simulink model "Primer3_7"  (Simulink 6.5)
settings: Solver=ode23t  StartTime=0.0  StopTime=5  RelTol=1e-3
undefined symbols (not defined in the file or in its folder): blocks, Continuous, powergui, ZData
libraries: powerlib x3, powerlib_extras x2

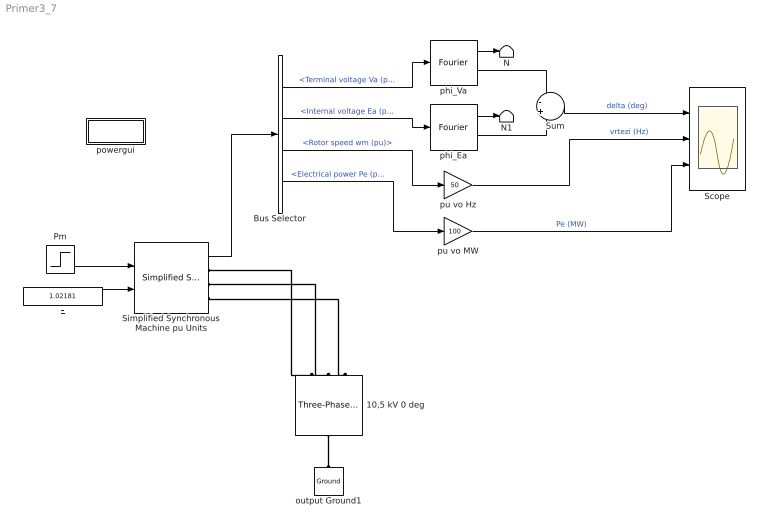
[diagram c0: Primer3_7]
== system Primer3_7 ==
  10,5 kV 0 deg : powerlib/Electrical Sources/Three-Phase Programmable Voltage Source  Orientation=up  DialogController=PMDialogs.PMDefaultMaskDlg  SystemSampleTime=-1  PositiveSequence="[10.5e3 0  50]"  VariationEntity=None  VariationType=Step  VariationStep=-0.5  VariationRate=10  VariationMagnitude=0.3  VariationFrequency=2  VariationTiming=[0.1 1.2]  VariationPhaseA=off  Amplitudes=[1 0.8 1.2 1.0]  TimeValues=[0 0.1 0.15 0.2]  HarmonicGeneration=off  HarmonicA=[3 0.2 -25 0]  HarmonicB="[2 0.15  35 2]"  Timing="[0.05  3]"
  Bus Selector : BusSelector  OutputSignals=Terminal voltage Va (pu),Internal voltage Ea (pu),Rotor speed wm (pu),Electrical power Pe (pu)
  E : Constant  Value=1.02181  OutDataType=sfix(16)  ConRadixGroup=Use specified scaling  OutScaling=2^0  SampleTime=inf  FramePeriod=inf
  N : Terminator
  N1 : Terminator
  Pm : Step  Time=0.5  Before=0.5  After=0.6  SampleTime=0
  Scope : Scope  NumInputPorts=3
  Simplified Synchronous Machine pu Units : powerlib/Machines/Simplified Synchronous Machine pu Units  DialogController=PMDialogs.PMDefaultMaskDlg  SystemSampleTime=-1  ConnectionType=3-wire Y  NominalParameters=[100e6 10.5e3 50]  Mechanical=[6 20 1]  InternalRL="[0  0.3+0.12]"  InitialConditions=[0 11.8598 0.5 0.5 0.5 0 -120 120]  Units=0  LoadFlowParameters=[1 50000000 0 0 0]
  Sum : Sum  Inputs=-+
  output Ground1 : powerlib/Elements/Ground  Orientation=down  DialogController=PMDialogs.PMDefaultMaskDlg  PhysicalDomain=powersysdomain  SubClassName=unknown  LeftPortType=p1  RightPortType=p1  LConnTagsString=a
  phi_Ea : powerlib_extras/Measurements/Fourier  DialogController=PMDialogs.PMDefaultMaskDlg  SystemSampleTime=-1  f1=50  n=1
  phi_Va : powerlib_extras/Measurements/Fourier  DialogController=PMDialogs.PMDefaultMaskDlg  SystemSampleTime=-1  f1=50  n=1
  powergui : Subsystem  AncestorBlock=powerlib/powergui  InitFcn=powergui( 'InitFcn_Callback' , gcb , 0 , [ ] );  mask(PSB option menu block){SimulationMode=Continuous, SampleTime=50e-6, echomessages=off, RestoreLinks=warning, x0status=blocks, Frange=[0:2:500], Ylog=off, Xlog=on, ShowGrid=off, save=off, variable=ZData, structure=, ZoomFFT=on, StartTime=0.0, cycles=1, DisplayStyle=1, fundamental=60, FreqAxis=off, MaxFrequency=1000, frequencyindice=50, frequencyindicesteady=1, RmsSteady=1, display=off, Ts=0, frequency=60, methode=off, HookPort=off, Interpol=off}
      mask prompts: SimulationMode "Simulation mode"; SampleTime "Sample time Ts (when simulation mode is Discrete) (s)"; echomessages "Echo  Messages"; RestoreLinks "Restore disabled links"; x0status "Initial electrical states status"; Frange "Impedance tool: Frequency Range"; Ylog "Impedance tool: Log impedance"; Xlog "Impedance tool: log Frequency"; ShowGrid "Impedance tool: grid"; save "Impedance tool: Save Data To Workspace"; variable "Impedance tool: Variable Name"; structure "Structure Name (PSBFFTSCOPE)"; ZoomFFT "ZoomFFT (PSBFFTSCOPE)"; StartTime "Start Time (PSBFFTSCOPE)"; cycles "Cycles (PSBFFTSCOPE)"; DisplayStyle "Display style (PSBFFTSCOPE)"; fundamental "Fundamental (PSBFFTSCOPE)"; FreqAxis "Frequency Axis (PSBFFTSCOPE)"; MaxFrequency "Max Frequency (PSBFFTSCOPE)"; frequencyindice "Load flow frequency (Hz)"; frequencyindicesteady "Frequency indice (STEADYSTATE)"; RmsSteady "RMS display (STEADYSTATE)"; display "Display Results"; Ts "OBSOLETE 1"; frequency "Phasor frequency (Hz)"; methode "Phasor simulation"; HookPort "Hook port"; Interpol "Interpolate"
      mask init:
      | powerlibroot = which('powersysdomain');
      | PSBroot = powerlibroot(1:end-16);
      | %
      | switch SimulationMode
      | 	case 1
      | 		message=sprintf('Continuous');
      | 	case 2
      |         SampleTimeeval=evalin('base',SampleTime,'NaN');
      |         if isnan(SampleTimeeval)
      |             message=sprintf('Warning !!,\nUndefined sample time');
      |         else
      |             message=sprintf('Discrete,\nTs = %.4g s.',SampleTimeeval);
      |         end
      | 	case 3
      | 		message=sprintf('Phasors');
      | end
      | if strcmp(bdroot,'powerlib')
      |   message='powergui';
      | end
      | power_initmask();
  pu vo Hz : Gain  Gain=50
  pu vo MW : Gain  Gain=100
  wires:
  E/1 -> Simplified Synchronous Machine pu Units/2
  Pm/1 -> Simplified Synchronous Machine pu Units/1
  phi_Va/2 -> Sum/1
  phi_Ea/2 -> Sum/2
  Sum/1 -> Scope/1  "delta (deg)"
  phi_Va/1 -> N/1
  phi_Ea/1 -> N1/1
  Bus Selector/1 -> phi_Va/1  "<Terminal voltage Va (pu)>"
  Bus Selector/2 -> phi_Ea/1  "<Internal voltage Ea (pu)>"
  Simplified Synchronous Machine pu Units/1 -> Bus Selector/1
  Bus Selector/3 -> pu vo Hz/1  "<Rotor speed wm (pu)>"
  pu vo Hz/1 -> Scope/2  "vrtezi (Hz)"
  Bus Selector/4 -> pu vo MW/1  "<Electrical power Pe (pu)>"
  pu vo MW/1 -> Scope/3  "Pe (MW)"
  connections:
  output Ground1/LConn1 -- 10,5 kV 0 deg/LConn1
  Simplified Synchronous Machine pu Units/RConn3 -- 10,5 kV 0 deg/RConn3
  Simplified Synchronous Machine pu Units/RConn2 -- 10,5 kV 0 deg/RConn2
  Simplified Synchronous Machine pu Units/RConn1 -- 10,5 kV 0 deg/RConn1

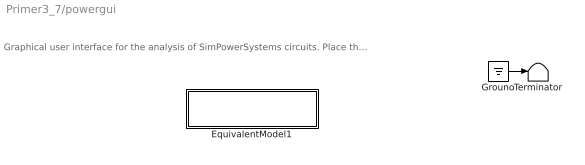
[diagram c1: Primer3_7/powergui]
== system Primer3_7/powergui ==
  note: Graphical user interface for the analysis of SimPowerSystems circuits. Place the Powergui block in the top-level of your model and double-click on it to open the GUI.
  EquivalentModel1 : Subsystem
  Ground : Ground
  Terminator : Terminator
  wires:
  Ground/1 -> Terminator/1

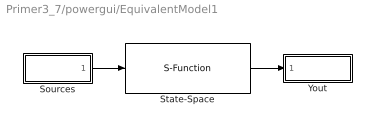
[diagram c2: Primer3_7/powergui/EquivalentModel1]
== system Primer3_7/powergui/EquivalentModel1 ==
  Sources : Subsystem
  State-Space : S-Function  FunctionName=sfun_spssw_contc  Parameters=A, B, C, D, x0
  Yout : Subsystem
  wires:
  State-Space/1 -> Yout/1(v,i)
  Sources/1(u) -> State-Space/1

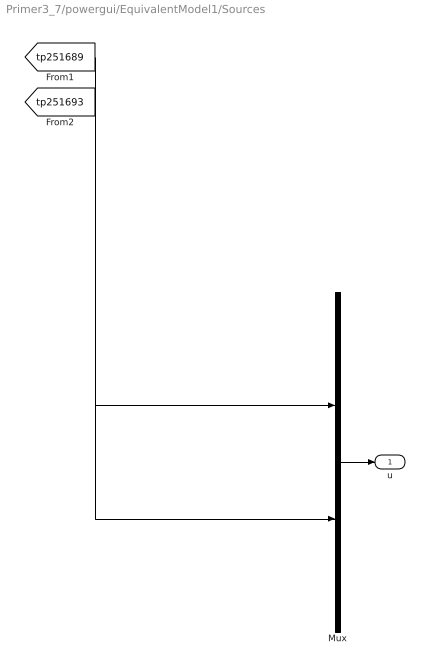
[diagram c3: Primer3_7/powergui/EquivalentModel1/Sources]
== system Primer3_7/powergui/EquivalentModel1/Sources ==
  Mux : Mux  Inputs=[2 3]
  u : Outport
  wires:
  Mux/1 -> u/1
  [tp251689] -> Mux/1
  [tp251693] -> Mux/2

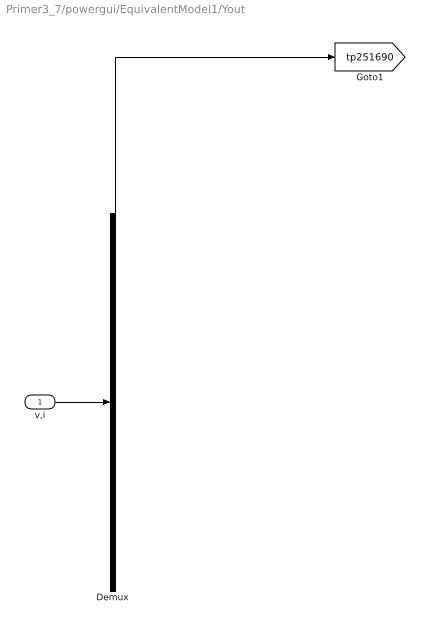
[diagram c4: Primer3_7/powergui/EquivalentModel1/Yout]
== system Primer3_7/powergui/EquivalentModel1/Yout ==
  v,i : Inport
  Demux : Demux  Outputs=1
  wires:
  v,i/1 -> Demux/1
  Demux/1 -> [tp251690]
